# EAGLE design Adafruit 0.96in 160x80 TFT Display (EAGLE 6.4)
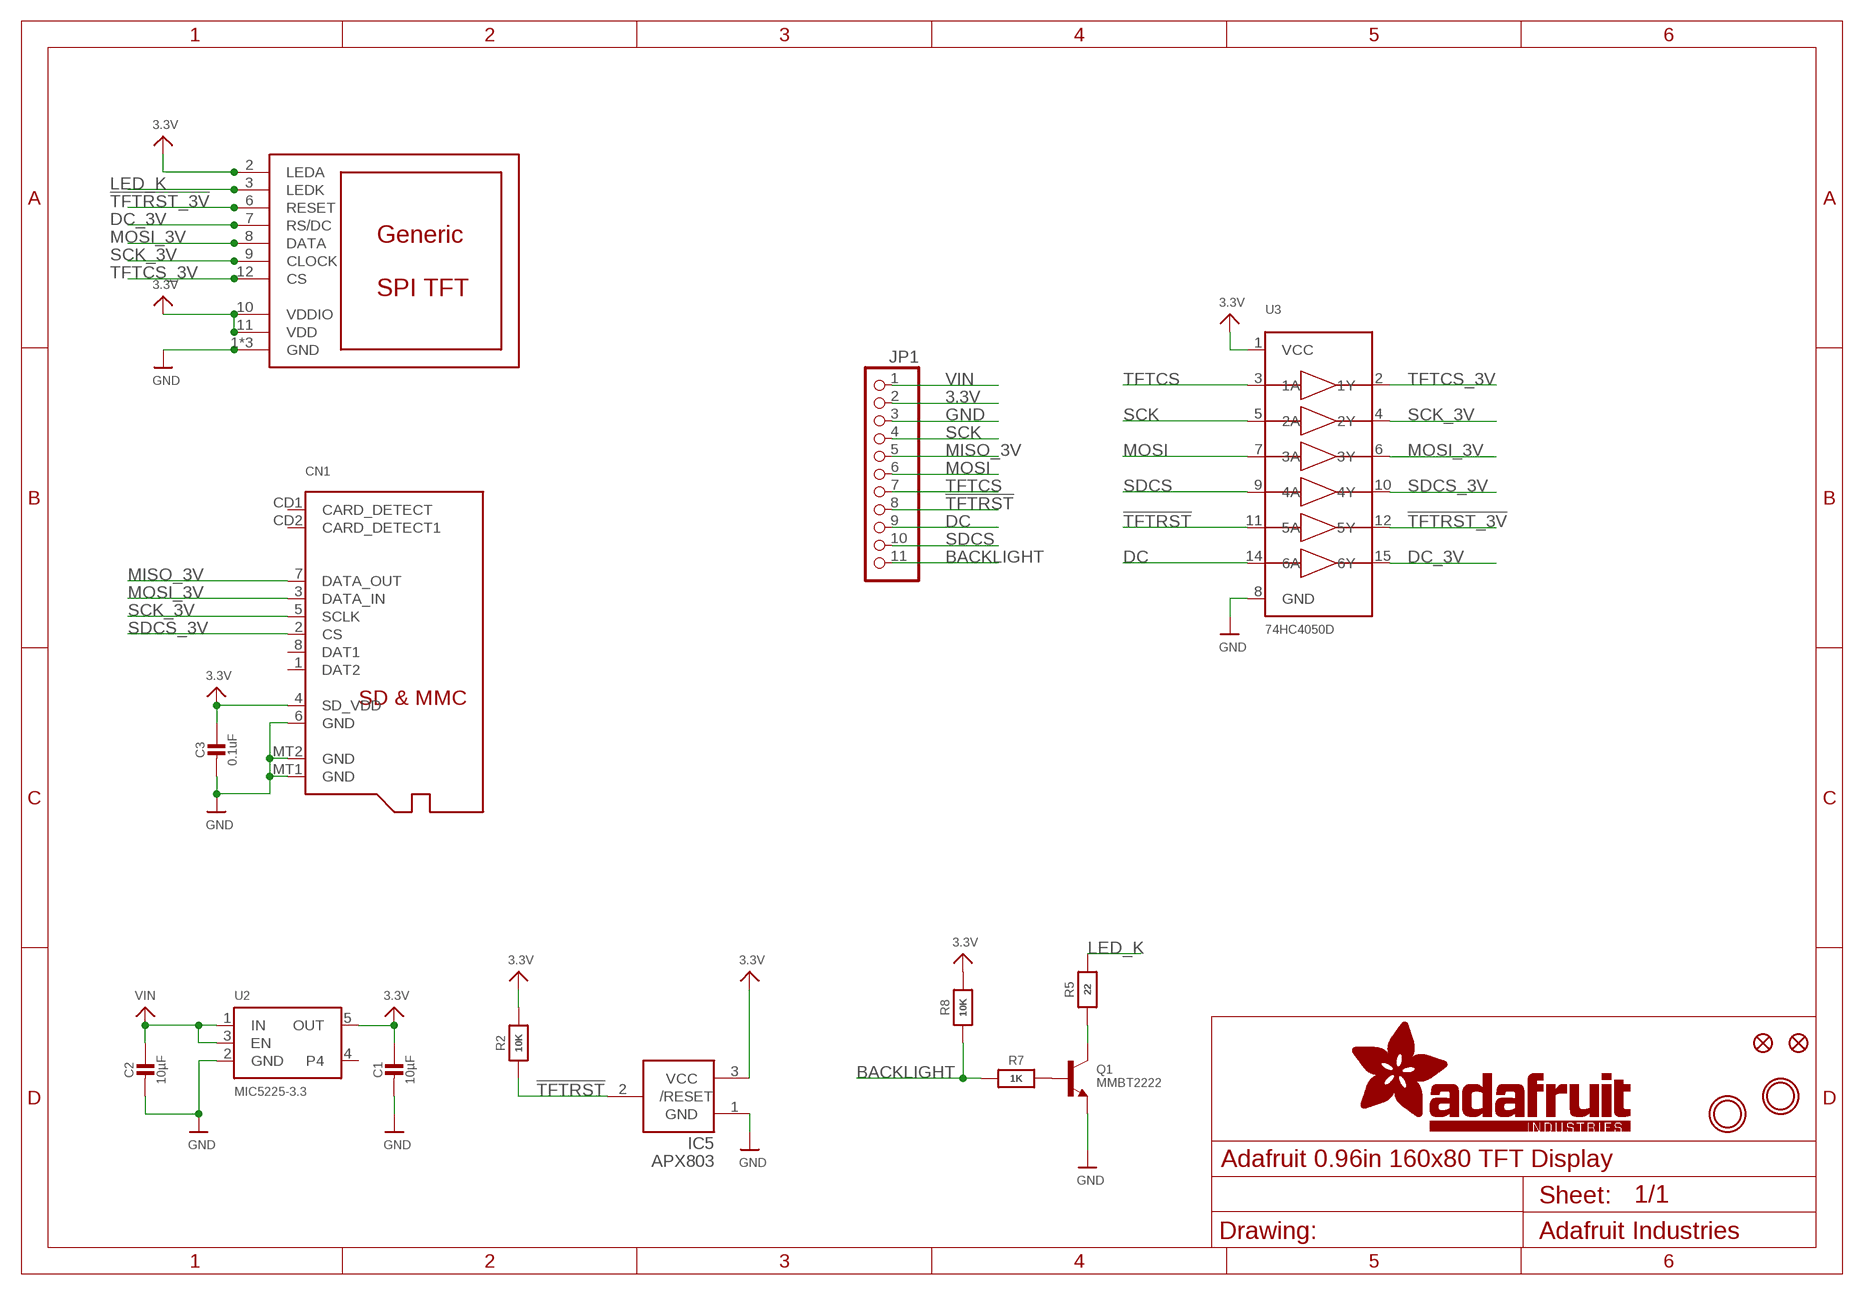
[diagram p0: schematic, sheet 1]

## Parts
C1  10µF  CAP_CERAMIC0805-NOOUTLINE  [0805-NO]
C2  10µF  CAP_CERAMIC0805-NOOUTLINE  [0805-NO]
C3  0.1uF  CAP_CERAMIC0805-NOOUTLINE  [0805-NO]
CN1  MICROSD  [MICROSD]
FID1  FIDUCIAL_1MM  [FIDUCIAL_1MM]
FID2  FIDUCIAL_1MM  [FIDUCIAL_1MM]
IC5  APX803  AXP083-SAG  [SOT23]
JP1  HEADER-1X11  [1X11_ROUND]
Q1  MMBT2222  TRANSISTOR_NPNWIDE  [SOT23-WIDE]
R2  10K  RESISTOR_0603_NOOUT  [0603-NO]
R5  22  RESISTOR_0603_NOOUT  [0603-NO]
R7  1K  RESISTOR_0603_NOOUT  [0603-NO]
R8  10K  RESISTOR_0603_NOOUT  [0603-NO]
U2  MIC5225-3.3  VREG_SOT23-5  [SOT23-5]
U3  74HC4050D  [SOIC16]
U$2  DISP_LCD_0.9IN_160X80  [TFT_0.96IN_160X80]
U$9  MOUNTINGHOLE2.5  [MOUNTINGHOLE_2.5_PLATED]
U$10  MOUNTINGHOLE2.5  [MOUNTINGHOLE_2.5_PLATED]

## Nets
3.3V: C1.1 C3.1 CN1.4(SD_VDD) IC5.3(VCC) JP1.2 R2.2 R8.2 U2.5(OUT) U3.1(VCC) U$2.2(LEDA) U$2.10(VDDIO) U$2.11(VDD)
!TFTRST: IC5.2(/RESET) JP1.8 R2.1 U3.11(5A)
!TFTRST_3V: U3.12(5Y) U$2.6(RESET)
BACKLIGHT: JP1.11 R7.1 R8.1
DC: JP1.9 U3.14(6A)
DC_3V: U3.15(6Y) U$2.7(RS/DC)
GND: C1.2 C2.2 C3.2 CN1.6(GND) CN1.MT1(GND) CN1.MT2(GND) IC5.1(GND) JP1.3 Q1.2(E) U2.2(GND) U3.8(GND) U$2.1(GND) U$2.5(GND) U$2.13(GND)
LED_K: R5.2 U$2.3(LEDK)
MISO_3V: CN1.7(DATA_OUT) JP1.5
MOSI: JP1.6 U3.7(3A)
MOSI_3V: CN1.3(DATA_IN) U3.6(3Y) U$2.8(DATA)
N$1: Q1.1(B) R7.2
N$5: Q1.3(C) R5.1
SCK: JP1.4 U3.5(2A)
SCK_3V: CN1.5(SCLK) U3.4(2Y) U$2.9(CLOCK)
SDCS: JP1.10 U3.9(4A)
SDCS_3V: CN1.2(CS) U3.10(4Y)
TFTCS: JP1.7 U3.3(1A)
TFTCS_3V: U3.2(1Y) U$2.12(CS)
VIN: C2.1 JP1.1 U2.1(IN) U2.3(EN)
Unconnected: CN1.1(DAT2) CN1.8(DAT1) CN1.CD1(CARD_DETECT) CN1.CD2(CARD_DETECT1) U2.4

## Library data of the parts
C1-C3 = microbuilder:CAP_CERAMIC: Ceramic Capacitors
CN1 = microbuilder:MICROSD: MicroSD/Transflash Card Holder with SPI pinout 3M: 2908-05WB-MG 4UConnector: 19656 Footprint courtesy: Adafruit Industries
FID1 FID2 = microbuilder:FIDUCIAL: Fiducial Alignment Points; BOM: EXCLUDE
IC5 = adafruit:AXP083
JP1 = microbuilder:HEADER-1X11
Q1 = microbuilder:TRANSISTOR_NPN: NPN Transistor Transistor (NPN) 500mA 45V - BC817 [Digikey: 568-1631-1-ND] Transistor (NPN) 500mA 45V - BC817,215 [Mouser: 771-BC817-T/R] SOT23-R - SOT23 footprint optimised for use with solder paste and reflow ovens. SOT23-W - SOT23 footprint optimised for hand-soldering (larger pads).
R2 R5 R7 R8 = microbuilder:RESISTOR: Resistors
U2 = microbuilder:VREG_SOT23-5: SOT23-5 Fixed Voltage Regulators Part Current Out V Out V In V Dropout θJA (°C/W) TJ (°C) Digikey Part No. ADP121 150mA 3.3V 3.4-5.5V 0.09V @ 150mA -- -- ADP121-AUJZ33R7CT-ND ADP121 150mA 3.0V 3.1-5.5V 0.09V @ 150mA -- -- ADP121-AUJZ30R7CT-ND ADP122 300mA 3.3V 3.4-5.5V 0.085V @ 300mA -- --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
U3 = microbuilder:74HC4050D: 6-channel level shifter 74HC4050D - 2V-6V Supply SOIC16 Digikey: 74HC4050D,653-ND Mouser: 771-74HC4050D-T TSSOP16 Digikey: 296-9215-1-ND Mouser:
U$2 = microbuilder:DISP_LCD_0.9IN_160X80
U$9 U$10 = microbuilder:MOUNTINGHOLE: Mounting Hole; BOM: EXCLUDE

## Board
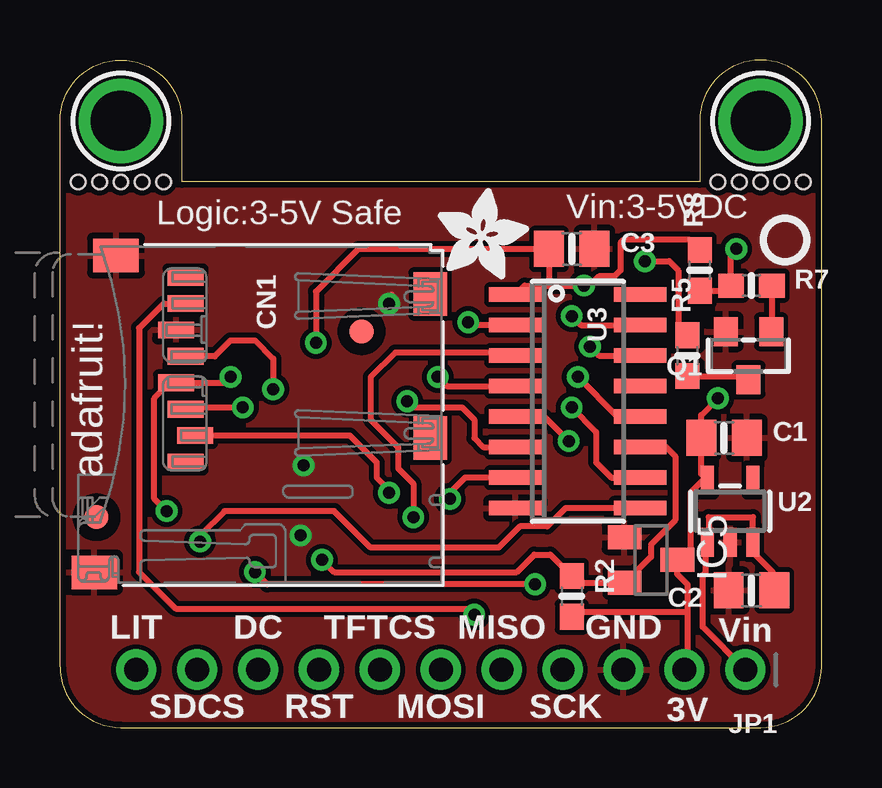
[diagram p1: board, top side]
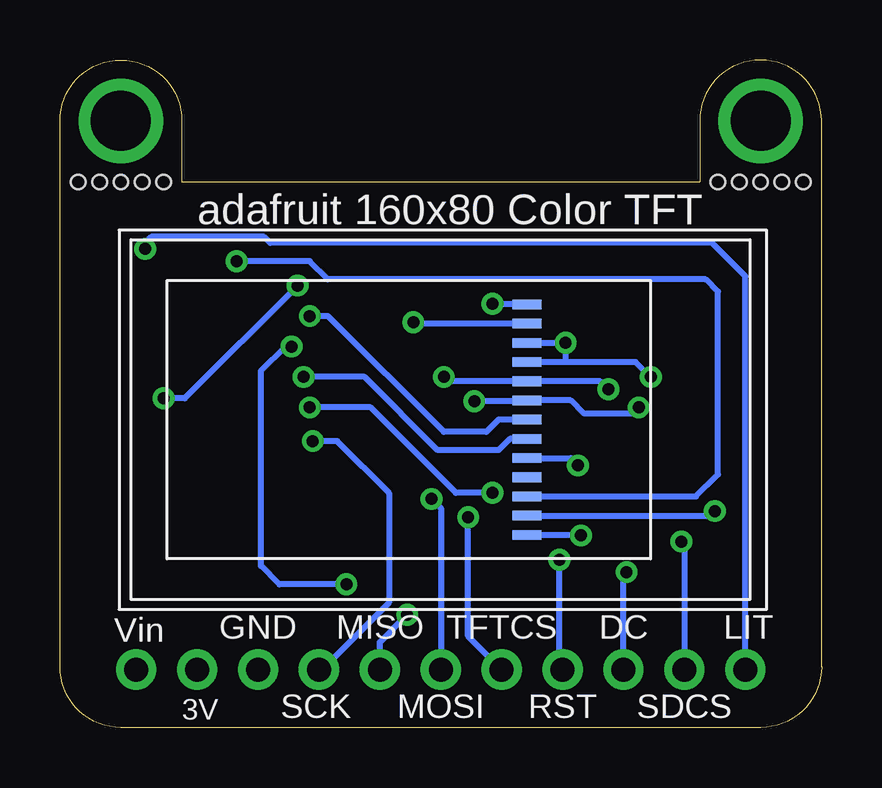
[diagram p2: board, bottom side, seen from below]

Size 31.75 x 27.81 mm. Coordinates in mm from the lower left corner, seen from the top.
Outline: 0,2.54 0,25.27 arc-90 2.54,27.81 arc-90 5.08,25.27 5.08,22.73 26.67,22.73 26.67,25.27 arc-90 29.21,27.81 arc-90 31.75,25.27 31.75,2.54 arc-90 29.21,0 2.54,0 arc-90 0,2.54
Copper layers (1*16): Top 0.035mm / dielectric 1.5mm / Bottom 0.035mm
Design rules "adafruit *": minimum track width 8mil, minimum drill 15.5mil, track to track 8mil, track to pad 8mil, pad to pad 8mil, via to via 8mil, smd to smd 8mil, copper to edge 10mil, drill to drill 8mil, minimum pad ring 10mil, minimum via ring 8mil, stop-mask expansion 2mil, vias tented up to drill 20mil, thermal gap 10mil
Holes 0.6 mm at 4.32,22.73 3.43,22.73 2.54,22.73 1.65,22.73 0.76,22.73 30.99,22.73 30.1,22.73 29.21,22.73 28.32,22.73 27.43,22.73

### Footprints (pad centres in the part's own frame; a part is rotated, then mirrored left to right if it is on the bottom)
0805-NO = smd 1.24 x 1.5: 1 -0.95,0; 2 0.95,0
MICROSD = smd 0.7 x 1.5: 1 9,-10.64; 2 7.9,-10.24; 3 6.8,-10.64; 4 5.7,-11.04; 5 4.6,-10.64; 6 3.5,-11.04; 7 2.4,-10.64; 8 1.3,-10.64 | smd 1.8 x 1.4: CD1 2,-0.44; CD2 8,-0.44 | smd 1.4 x 1.9: MT1 0.4,-13.54; MT2 13.6,-14.44
FIDUCIAL_1MM = smd 1 x 1: 1 0,0
SOT23 = smd 1 x 1.4: 1 -0.95,-1.1; 2 0.95,-1.1; 3 0,1.1
1X11_ROUND = drill 1 pad 1.676: 1 -12.7,0; 2 -10.16,0; 3 -7.62,0; 4 -5.08,0; 5 -2.54,0; 6 0,0; 7 2.54,0; 8 5.08,0; 9 7.62,0; 10 10.16,0; 11 12.7,0
SOT23-WIDE = smd 1 x 1.2: 1 -0.95,-1; 2 0.95,-1; 3 0,1
0603-NO = smd 1.075 x 1: 1 -0.85,0; 2 0.85,0
SOT23-5 = smd 0.55 x 1.2: 1 -0.95,-1.3; 2 0,-1.3; 3 0.95,-1.3; 4 0.95,1.3; 5 -0.95,1.3
SOIC16 = smd 0.6 x 2.2: 1 -4.445,-2.6; 2 -3.175,-2.6; 3 -1.905,-2.6; 4 -0.635,-2.6; 5 0.635,-2.6; 6 1.905,-2.6; 7 3.175,-2.6; 8 4.445,-2.6; 9 4.445,2.6; 10 3.175,2.6; 11 1.905,2.6; 12 0.635,2.6; 13 -0.635,2.6; 14 -1.905,2.6; 15 -3.175,2.6; 16 -4.445,2.6
TFT_0.96IN_160X80 = smd 0.4 x 1.2: 1 -4.8,10; 2 -4,10; 3 -3.2,10; 4 -2.4,10; 5 -1.6,10; 6 -0.8,10; 7 0,10; 8 0.8,10; 9 1.6,10; 10 2.4,10; 11 3.2,10; 12 4,10; 13 4.8,10
MOUNTINGHOLE_2.5_PLATED = drill 2.5 pad 3.2: P$1 0,0

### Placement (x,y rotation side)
C1  27.69,12.06 0 top
C2  28.83,5.71 180 top
C3  21.34,19.94 0 top
CN1  15.88,20.07 270 top
FID1  1.52,8.76 0 top
FID2  12.57,16.51 0 top
IC5  24.64,6.98 270 top
JP1  15.88,2.41 180 top
Q1  28.7,15.49 180 top
R2  21.34,5.46 270 top
R5  26.16,15.49 90 top
R7  28.83,18.41 0 top
R8  26.67,19.05 90 top
U2  27.94,9.02 0 top
U3  21.59,13.59 270 top
U$2  2.29,12.83 90 bottom
U$4  MICROSD  [ADAFRUIT_3.5MM]  15.75,18.67 0 top
U$6  [PCBFEAT-REV-040]  30.23,20.32 0 top
U$9  2.54,25.27 0 top
U$10  29.21,25.27 0 top

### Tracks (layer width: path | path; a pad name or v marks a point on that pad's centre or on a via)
3.3V  (via drill 0.5)
  Top 0.254: v10.67,16.03 10.67,18.16 12.45,19.94 C3.1 20.39,18.41 | 18.29,18.16 19.12,18.16 U3.1 19.37,18.41 20.39,18.41 | 26.16,4.83 26.16,5.97 25.74,6.39 IC5.3 26.29,6.98 26.29,9.78 26.83,10.32 U2.5 26.74,10.57 C1.1 26.74,13.02 v27.43,13.72 | 26.16,4.83 26.16,2.54 JP1.2 | 20.39,18.41 v21.84,18.41 | v4.45,9.02 3.94,9.53 3.94,13.72 4.59,14.37 CN1.4 6.87,14.37 v7.11,14.61 | R8.2 26.25,20.32 23.5,20.32 23.37,20.19 23.37,19.05 23.11,18.8 22.48,18.8 22.1,18.41 v21.84,18.41 | 26.16,4.83 21.55,4.83 R2.2 | 21.84,18.67 v21.84,18.41
  Bottom 0.254: 10.67,15.23 7.76,15.23 7.14,14.61 v7.11,14.61 | 10.67,15.23 U$2.10 | U$2.11 v10.67,16.03 10.67,15.23 | v21.84,18.41 26.54,13.72 v27.43,13.72 | U$2.2 4.63,8.83 v4.45,9.02
!TFTRST  (via drill 0.5)
  Top 0.254: v10.92,6.98 11.43,6.48 19.05,6.48 19.77,7.2 20.45,7.2 R2.1 21.61,6.04 IC5.2 23.56,6.04 24.64,7.11 24.64,7.62 25.65,8.64 25.65,11.3 25.27,11.68 U3.11 24.13,11.68
  Bottom 0.254: JP1.8 10.92,2.54 v10.92,6.98
!TFTRST_3V  (via drill 0.5)
  Top 0.254: v21.59,14.61 23.24,12.95 U3.12
  Bottom 0.254: U$2.6 12.99,12.03 13.46,11.56 16,11.56 19.05,14.61 v21.59,14.61
BACKLIGHT  (via drill 0.5)
  Top 0.254: R8.1 27.76,18.2 R7.1 27.98,19.72 v28.19,19.94
  Bottom 0.254: JP1.11 3.17,18.8 4.57,20.19 22.99,20.19 23.24,20.45 27.94,20.45 28.19,20.19 v28.19,19.94
DC  (via drill 0.5)
  Top 0.254: v19.81,5.97 8.64,5.97 v8.13,6.48 | v22.1,15.88 22.48,15.49 U3.14
  Bottom 0.254: v22.1,15.88 22.35,15.88 23.37,14.86 23.37,6.73 22.61,5.97 v19.81,5.97 | JP1.9 8.25,6.35 v8.13,6.48
DC_3V  (via drill 0.5)
  Top 0.254: v21.34,17.14 21.72,16.76 U3.15
  Bottom 0.254: U$2.7 13.46,12.83 13.97,12.32 15.75,12.32 20.57,17.14 v21.34,17.14
GND  (via drill 0.5)
  Top 0.254: v13.72,17.65 13.72,17.91 13.84,18.03
  Bottom 0.254: U$2.5 10.46,11.23 v10.16,10.92 | U$2.13 13.69,17.63 v13.72,17.65 | U$2.1 10.06,8.03 v10.03,8
  pour Top: 0,22.73 0,0 31.75,0 31.75,22.73
LED_K  (via drill 0.5)
  Top 0.254: v24.38,19.43 25.4,19.43 25.78,19.05 25.78,16.76 26.2,16.34 R5.2
  Bottom 0.254: U$2.3 5.23,9.63 4.32,10.54 4.32,18.16 4.83,18.67 20.57,18.67 21.34,19.43 v24.38,19.43
MISO_3V  (via drill 0.5)
  Top 0.254: v17.27,4.7 17.27,4.95 4.83,4.95 3.3,6.48 3.3,16.64 4.33,17.67 CN1.7
  Bottom 0.254: JP1.5 18.41,3.56 v17.27,4.7
MOSI  (via drill 0.5)
  Top 0.254: U3.7 16.89,10.41 16.26,9.78 v16.26,9.53
  Bottom 0.254: v16.26,9.53 15.88,9.14 JP1.6
MOSI_3V  (via drill 0.5)
  Top 0.254: v14.48,13.59 14.73,13.34 16.76,13.34 17.27,12.83 17.27,12.06 17.65,11.68 U3.6 | CN1.3 5.3,13.34 v7.62,13.34
  Bottom 0.254: v7.62,13.34 7.87,13.08 9.91,13.08 10.45,13.63 U$2.8 12.32,13.59 v14.48,13.59
N$1
  Top 0.254: R7.2 29.68,16.52 Q1.1
N$5
  Top 0.254: R5.1 28.55,14.64 Q1.3
SCK  (via drill 0.5)
  Top 0.254: U3.5 20.19,12.95 v21.21,11.94
  Bottom 0.254: v21.21,11.94 20.19,11.94 18.03,9.78 18.03,5.21 20.83,2.41 JP1.4
SCK_3V  (via drill 0.5)
  Top 0.254: v8.89,14.1 8.89,15.37 8.13,16.13 7.11,16.13 6.45,15.47 CN1.5 | v15.75,14.61 16.13,14.22 U3.4
  Bottom 0.254: v8.89,14.1 9.22,14.43 U$2.9 15.57,14.43 v15.75,14.61
SDCS  (via drill 0.5)
  Top 0.254: U3.9 21.08,9.14 20.32,8.38 19.18,8.38 18.29,7.49 12.95,7.49 11.43,9.02 6.86,9.02 5.84,8 v5.84,7.75
  Bottom 0.254: v5.84,7.75 5.71,7.62 JP1.10
SDCS_3V  (via drill 0.5)
  Top 0.254: v21.34,13.34 22.35,12.32 22.35,11.05 22.99,10.41 U3.10 | v13.72,9.78 13.72,9.91 13.21,10.41 13.21,11.05 12.09,12.17 CN1.2
  Bottom 0.254: v13.72,9.78 15.24,9.78 18.8,13.34 v21.34,13.34
TFTCS  (via drill 0.5)
  Top 0.254: U3.3 18.99,15.62 13.97,15.62 12.95,14.61 12.95,12.83 14.1,11.68 14.1,10.79 14.73,10.16 v14.73,8.76
  Bottom 0.254: JP1.7 14.73,3.81 v14.73,8.76
TFTCS_3V  (via drill 0.5)
  Top 0.254: U3.2 17.14,16.76 v17.02,16.89
  Bottom 0.254: U$2.12 16.95,16.83 v17.02,16.89
VIN
  Top 0.254: JP1.1 26.8,4.19 26.8,6.35 26.92,6.48 26.92,7.65 U2.1 27.05,7.78 27.05,8.76 28.89,8.76 U2.3 28.89,7.3 29.72,6.48 29.72,5.78 C2.1

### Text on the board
tPlace: Logic:3-5V Safe | Vin:3-5VDC | adafruit! | LIT | DC | TFTCS | MISO | GND | Vin | SDCS | RST | MOSI | SCK | 3V
bPlace: adafruit 160x80 Color TFT | LIT | DC | TFTCS | MISO | GND | Vin | SDCS | RST | MOSI | SCK | 3V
